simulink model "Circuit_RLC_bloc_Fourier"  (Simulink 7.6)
settings: Solver=ode23t  StartTime=0.0  StopTime=0.02  RelTol=1e-3
InitFcn:
  | clc
StopFcn:
  | load Ampl_Phase_VC1.mat
  | plot(x(1,:),x(2,:),x(1,:),x(3,:))
  | grid
  | axis([0 0.02 -150 150])
  | title('Amplitude et phase _ Vc1')
  | xlabel('temps')
  | 
  | figure
  | 
  | load Ampl_Phase_VC2.mat
  | plot(y(1,:),y(2,:),y(1,:),y(3,:))
  | grid
  | axis([0 0.02 -150 150])
  | title('Amplitude et phase - Vc2')
  | xlabel('temps')
libraries: powerlib x11, powerlib_extras x2

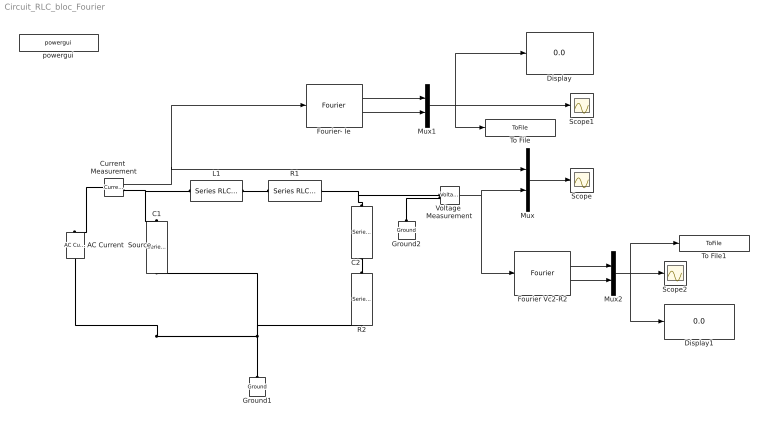
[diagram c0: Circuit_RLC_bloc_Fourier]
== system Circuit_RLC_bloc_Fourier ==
  AC Current  Source : powerlib/Electrical Sources/AC Current Source  DialogController=POWERSYS.PowerSysDialog  SystemSampleTime=-1  Amplitude=100  Phase=-30  Frequency=1000/(2*pi)  SampleTime=0  Measurements=None
  C1 : powerlib/Elements/Series RLC Branch  DialogController=POWERSYS.PowerSysDialog  PhysicalDomain=powersysdomain  SubClassName=unknown  LeftPortType=p1  RightPortType=p1  LConnTagsString=__new0  RConnTagsString=__new0  BranchType=C  Resistance=1  Inductance=1e-3  SetiL0=off  InitialCurrent=0  Capacitance=0.001  Setx0=off  InitialVoltage=0  Measurements=None
  C2 : powerlib/Elements/Series RLC Branch  DialogController=POWERSYS.PowerSysDialog  PhysicalDomain=powersysdomain  SubClassName=unknown  LeftPortType=p1  RightPortType=p1  LConnTagsString=__new0  RConnTagsString=__new0  BranchType=C  Resistance=1  Inductance=1e-3  SetiL0=off  InitialCurrent=0  Capacitance=0.001  Setx0=off  InitialVoltage=0  Measurements=None
  Current  Measurement : powerlib/Measurements/Current Measurement  DialogController=POWERSYS.PowerSysDialog  SystemSampleTime=-1  PhasorSimulation=off  OutputType=Complex  PSBequivalent=0
  Display : Display
  Display1 : Display
  Fourier Vc2-R2 : powerlib_extras/Measurements/Fourier  DialogController=POWERSYS.PowerSysDialog  SystemSampleTime=-1  f1=1000/(2*pi)  n=1
  Fourier- Ie : powerlib_extras/Measurements/Fourier  DialogController=POWERSYS.PowerSysDialog  SystemSampleTime=-1  f1=1000/(2*pi)  n=1
  Ground1 : powerlib/Elements/Ground  DialogController=POWERSYS.PowerSysDialog  PhysicalDomain=powersysdomain  SubClassName=unknown  LeftPortType=p1  RightPortType=p1  LConnTagsString=a
  Ground2 : powerlib/Elements/Ground  DialogController=POWERSYS.PowerSysDialog  PhysicalDomain=powersysdomain  SubClassName=unknown  LeftPortType=p1  RightPortType=p1  LConnTagsString=a
  L1 : powerlib/Elements/Series RLC Branch  DialogController=POWERSYS.PowerSysDialog  PhysicalDomain=powersysdomain  SubClassName=unknown  LeftPortType=p1  RightPortType=p1  LConnTagsString=__new0  RConnTagsString=__new0  BranchType=L  Resistance=4  Inductance=1e-3  SetiL0=off  InitialCurrent=0  Capacitance=0  Setx0=off  InitialVoltage=0  Measurements=None
  Mux : Mux  Inputs=2
  Mux1 : Mux  Inputs=2
  Mux2 : Mux  Inputs=2
  R1 : powerlib/Elements/Series RLC Branch  DialogController=POWERSYS.PowerSysDialog  PhysicalDomain=powersysdomain  SubClassName=unknown  LeftPortType=p1  RightPortType=p1  LConnTagsString=__new0  RConnTagsString=__new0  BranchType=R  Resistance=1  Inductance=10e-3  SetiL0=off  InitialCurrent=0  Capacitance=0  Setx0=off  InitialVoltage=0  Measurements=None
  R2 : powerlib/Elements/Series RLC Branch  DialogController=POWERSYS.PowerSysDialog  PhysicalDomain=powersysdomain  SubClassName=unknown  LeftPortType=p1  RightPortType=p1  LConnTagsString=__new0  RConnTagsString=__new0  BranchType=R  Resistance=1  Inductance=10e-3  SetiL0=off  InitialCurrent=0  Capacitance=0  Setx0=off  InitialVoltage=0  Measurements=None
  Scope : Scope
  Scope1 : Scope
  Scope2 : Scope
  To File : ToFile  Filename=Ampl_Phase_VC1  MatrixName=x
  To File1 : ToFile  Filename=Ampl_Phase_VC2  MatrixName=y
  Voltage  Measurement : powerlib/Measurements/Voltage Measurement  DialogController=POWERSYS.PowerSysDialog  SystemSampleTime=-1  PhasorSimulation=off  OutputType=Complex  PSBequivalent=0
  powergui : powerlib/powergui  Priority=1  SystemSampleTime=-1  SimulationMode=Continuous  SampleTime=50e-6  frequency=60  SPID=off  DisableSnubberDevices=off  DisableRonSwitches=off  DisableVfSwitches=off  SwTol=0  Interpol=off  frequencyindice=159.154943091895  echomessages=off  HookPort=off  DisplayEquations=off  FunctionMessages=off  EnableUseOfTLC=off  x0status=blocks  RestoreLinks=warning  ResistiveCurrentMeasurement=off  Frange=[0:2:500]  Ylog=off  Xlog=on  ShowGrid=on  save=off  variable=ZData  ZoomFFT=off  StartTime=0.0  cycles=1  DisplayStyle=1  fundamental=60  FreqAxis=off  MaxFrequency=1000  frequencyindicesteady=1  display=off  methode=off
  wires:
  Voltage  Measurement/1 -> Mux/2, Fourier Vc2-R2/1
  Mux/1 -> Scope/1
  Current  Measurement/1 -> Mux/1, Fourier- Ie/1
  Fourier- Ie/1 -> Mux1/1
  Fourier- Ie/2 -> Mux1/2
  Mux1/1 -> Scope1/1, Display/1, To File/1
  Mux2/1 -> Scope2/1, Display1/1, To File1/1
  Fourier Vc2-R2/1 -> Mux2/1
  Fourier Vc2-R2/2 -> Mux2/2
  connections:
  Current  Measurement/RConn1 -- C1/LConn1 -- L1/LConn1
  AC Current  Source/LConn1 -- C1/RConn1 -- R2/LConn1 -- Ground1/LConn1
  Ground2/LConn1 -- Voltage  Measurement/LConn2
  Current  Measurement/LConn1 -- AC Current  Source/RConn1
  C2/LConn1 -- R1/RConn1 -- Voltage  Measurement/LConn1
  R1/LConn1 -- L1/RConn1
  C2/RConn1 -- R2/RConn1
